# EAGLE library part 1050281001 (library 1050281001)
CONN CAM SOCKET 32POS GOLD Source: Datasheet
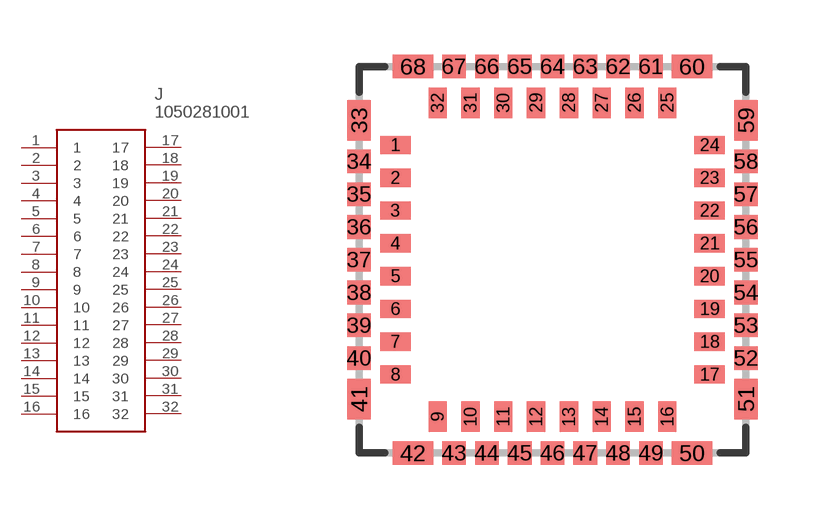
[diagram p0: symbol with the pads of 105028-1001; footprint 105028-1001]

Designator prefix J

## 1050281001 (Arrow_Part_Number: 1050281001; Arrow_Price-Stock: https://www.arrow.com/en/products/1050281001/molex?utm_currency=USD&region=nac; Description: CONN CAM SOCKET 32POS GOLD; Height: mm; Manufacturer_Name: Molex; Manufacturer_Part_Number: 1050281001)  [105028-1001]
1  1
2  2
3  3
4  4
5  5
6  6
7  7
8  8
9  9
10  10
11  11
12  12
13  13
14  14
15  15
16  16
17  17
18  18
19  19
20  20
21  21
22  22
23  23
24  24
25  25
26  26
27  27
28  28
29  29
30  30
31  31
32  32

## Footprint 105028-1001 (pad centres in mm)
105028-1001
smd 0.84 x 0.5: 1 -4.31,3.15; 2 -4.31,2.25; 3 -4.31,1.35; 4 -4.31,0.45; 5 -4.31,-0.45; 6 -4.31,-1.35; 7 -4.31,-2.25; 8 -4.31,-3.15; 17 4.31,-3.15; 18 4.31,-2.25; 19 4.31,-1.35; 20 4.31,-0.45; 21 4.31,0.45; 22 4.31,1.35; 23 4.31,2.25; 24 4.31,3.15
smd 0.5 x 0.84: 9 -3.15,-4.31; 10 -2.25,-4.31; 11 -1.35,-4.31; 12 -0.45,-4.31; 13 0.45,-4.31; 14 1.35,-4.31; 15 2.25,-4.31; 16 3.15,-4.31; 25 3.15,4.31; 26 2.25,4.31; 27 1.35,4.31; 28 0.45,4.31; 29 -0.45,4.31; 30 -1.35,4.31; 31 -2.25,4.31; 32 -3.15,4.31
smd 0.65 x 1.1: 33 -5.305,3.825; 41 -5.305,-3.825; 51 5.305,-3.825; 59 5.305,3.825
smd 0.65 x 0.65: 34 -5.305,2.7; 35 -5.305,1.8; 36 -5.305,0.9; 37 -5.305,0; 38 -5.305,-0.9; 39 -5.305,-1.8; 40 -5.305,-2.7; 43 -2.7,-5.305; 44 -1.8,-5.305; 45 -0.9,-5.305; 46 0,-5.305; 47 0.9,-5.305; 48 1.8,-5.305; 49 2.7,-5.305; 52 5.305,-2.7; 53 5.305,-1.8; 54 5.305,-0.9; 55 5.305,0; 56 5.305,0.9; 57 5.305,1.8; 58 5.305,2.7; 61 2.7,5.305; 62 1.8,5.305; 63 0.9,5.305; 64 0,5.305; 65 -0.9,5.305; 66 -1.8,5.305; 67 -2.7,5.305
smd 1.1 x 0.65: 42 -3.825,-5.305; 50 3.825,-5.305; 60 3.825,5.305; 68 -3.825,5.305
